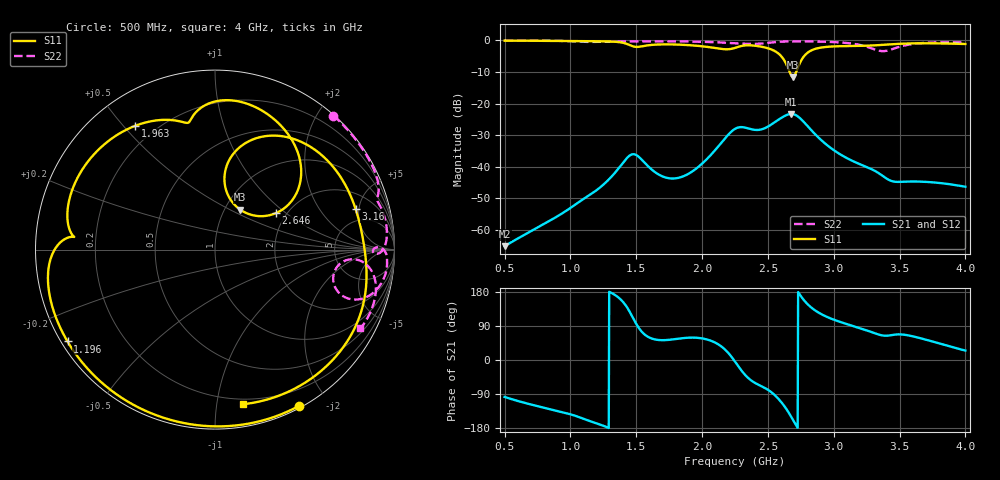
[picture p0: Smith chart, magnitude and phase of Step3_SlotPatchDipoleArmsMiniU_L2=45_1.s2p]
! TOUCHSTONE file generated by CST MICROWAVE STUDIO
! Date and time: Tue May 19 01:37:20 2020
! Project name: DualBand_DualMode_Antenna_FD_SteppedDesign.cst
! Parameters = {FPL=20; FPW=20; L=50; ST=10; SW=30; W=52; WF=7; ext=10; gap=1; inset=13}
! Header version: 2015
! Port assignment regex: !\s*Touchstone port\s*([0-9]+)\s*=\s*CST MWS port\s*([0-9]+)\s*\(\"(.*)\"\)(\s*mode\s*([0-9]+))?.*
! Touchstone port assignment:
! Touchstone port 1 = CST MWS port 1 ("")
! Touchstone port 2 = CST MWS port 2 ("")
# GHz S MA R 50
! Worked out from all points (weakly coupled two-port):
!   1006 points, 500 MHz to 4 GHz, reference 50 ohm
!   highest |S21| = -23.28 dB at 2.677 GHz (marker M1); lowest = -65.1 dB at 500 MHz (marker M2)
!   lowest |S11| = -11.6 dB at 2.691 GHz (marker M3), VSWR 1.71, Z = 59 + j28.2 ohm
!   |S11| at or under -10 dB: 2.665 GHz to 2.715 GHz (49.81 MHz wide, 1.85 % of centre)
!   |S22| runs from -3.4 to 0.0 dB; largest |S21 - S12| = 3.3e-05
!   S11 on the Smith chart (normalised r, x): 500 MHz: 0.02, -1.67; 1.196 GHz: 0.02, -0.29; 1.963 GHz: 0.13, +0.54; 2.646 GHz: 1.76, +0.85; 3.16 GHz: 3.42, +4.61; 4 GHz: 0.16, -1.18
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0.5  0.9887 -61.7  0.0005551 -97.4  0.0005551 -97.4  0.9964 48.5
0.787  0.9828 -97.0  0.001204 -125.0  0.001204 -125.0  0.9932 28.8
1.0845  0.9726 -133.8  0.002957 -153.2  0.002956 -153.2  0.9505 17.7
1.1965  0.9681 -148.1  0.004234 -166.9  0.004234 -166.9  0.9463 16.2
1.3575  0.9435 -170.6  0.008996 166.9  0.008995 166.9  0.9574 13.2
1.4695  0.8115 175.1  0.01575 114.8  0.01575 114.8  0.9611 11.1
1.669  0.8601 159.7  0.007575 52.8  0.007575 52.8  0.964 7.4
1.809  0.8582 141.9  0.006614 55.8  0.006614 55.8  0.9611 4.9
1.963  0.8203 122.8  0.009636 58.6  0.009636 58.6  0.9524 2.2
2.25  0.76 99.0  0.03981 -4.1  0.03981 -4.1  0.8988 -1.5
2.369  0.8347 79.4  0.03949 -52.9  0.03949 -52.9  0.8802 -0.7
2.5195  0.7268 51.9  0.04574 -83.3  0.04571 -83.3  0.9224 0.6
2.6455  0.3946 30.9  0.06636 -132.1  0.06636 -132.1  0.9592 -2.8
2.677  0.2787 44.2  0.06858 -149.9  0.06858 -149.9  0.9605 -3.6
2.691  0.2633 57.8  0.06814 -158.3  0.06814 -158.3  0.9609 -4.0
2.747  0.4562 82.4  0.05792 170.1  0.05792 170.1  0.9625 -5.3
2.8345  0.7009 64.8  0.03697 137.0  0.03697 137.0  0.9606 -7.7
2.978  0.7978 39.3  0.01979 109.4  0.01979 109.4  0.9437 -11.7
3.16  0.8154 16.1  0.01191 88.4  0.01191 88.4  0.8764 -17.9
3.419  0.8615 -11.7  0.006201 64.6  0.006225 64.7  0.698 -6.7
3.664  0.8987 -41.0  0.005821 57.0  0.005817 57.0  0.9043 -10.3
4  0.8754 -79.9  0.004835 25.0  0.004835 25.0  0.9217 -28.4
